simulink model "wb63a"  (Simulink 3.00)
settings: Solver=ode113  SolverMode=SingleTasking  StartTime=0.0  StopTime=30  RelTol=1e-3  AbsTol=1e-6
libraries: simulink_extras x1

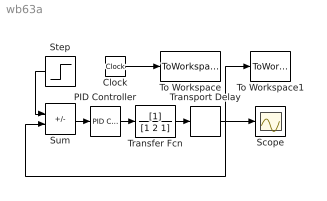
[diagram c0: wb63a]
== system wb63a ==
  Clock : Clock
  PID Controller : simulink_extras/Additional Linear/PID Controller  P=1.63488  I=1.63488/.9997325  D=1.63488*0.191767
  Scope : Scope
  Step : Step  Orientation=left  Time=0  Before=0  After=1  SampleTime=0
  Sum : Sum  Inputs=+-  SaturateOnIntegerOverflow=on
  To Workspace : ToWorkspace  VariableName=t  SampleTime=-1  SaveFormat=Matrix
  To Workspace1 : ToWorkspace  VariableName=y  SampleTime=-1  SaveFormat=Matrix
  Transfer Fcn : TransferFcn  Numerator=[1]  Denominator=[1 2 1]
  Transport Delay : TransportDelay  DelayTime=.5  InitialInput=0  BufferSize=1024
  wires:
  PID Controller/1 -> Transfer Fcn/1
  Sum/1 -> PID Controller/1
  Transport Delay/1 -> Scope/1, Sum/2, To Workspace1/1
  Transfer Fcn/1 -> Transport Delay/1
  Clock/1 -> To Workspace/1
  Step/1 -> Sum/1
